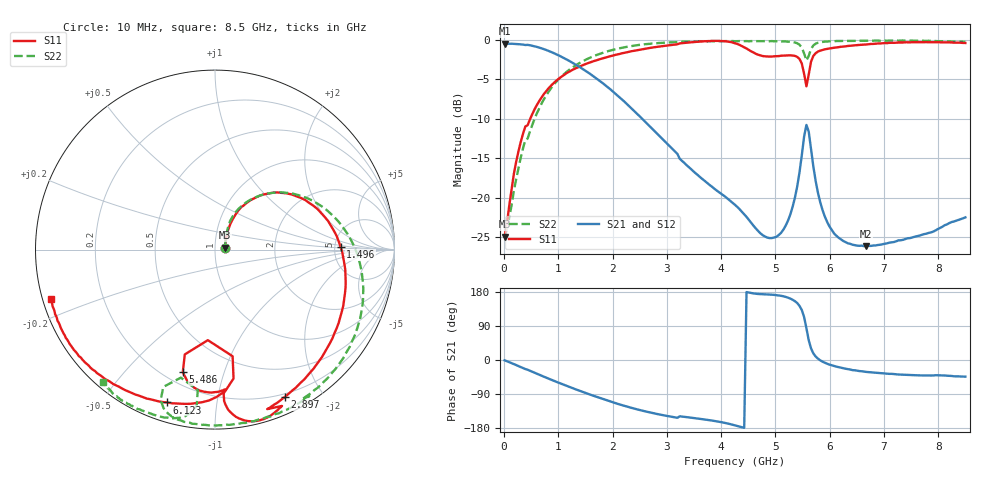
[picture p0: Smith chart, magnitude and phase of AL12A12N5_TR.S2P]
!AVX CORPORATION
!PART NUMBER AL12A12N5_TR
!DESCRIPTION: AIR CORE INDUCTOR, 12.5nH, 4 TURNS
!Agilent Technologies,E5071C,MY46102230,A.09.54
!Date: Mon Sep 03 15:48:47 2012
!Data & Calibration Information:
!Freq	S11:SOLT2(ON)	S21:SOLT2(ON)	S12:SOLT2(ON)	S22:SOLT2(ON)
# Hz S RI R 50
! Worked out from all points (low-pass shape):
!   201 points, 10 MHz to 8.5 GHz, reference 50 ohm
!   highest |S21| = -0.50 dB at 10 MHz (marker M1); lowest = -26.2 dB at 6.675 GHz (marker M2)
!   |S21| within 3 dB of the highest: start of sweep to 1.4 GHz
!   lowest |S11| = -25.0 dB at 10 MHz (marker M3), VSWR 1.12, Z = 55.9 + j1.16 ohm
!   |S11| at or under -10 dB: start of sweep to 483.2 MHz
!   |S22| runs from -24.9 to -0.1 dB; largest |S21 - S12| = 0.02
!   S11 on the Smith chart (normalised r, x): 10 MHz: 1.12, +0.02; 1.496 GHz: 5.64, +0.35; 2.897 GHz: 0.17, -1.56; 5.486 GHz: 0.27, -0.74; 6.123 GHz: 0.09, -0.73; 8.5 GHz: 0.02, -0.15
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1e7  0.0555 0.0103  0.9443 -0.0144  0.9353 0.00333  0.056 0.00982
1.798e8  0.0763 0.1184  0.9239 -0.1759  0.9254 -0.1758  0.0642 0.0892
3.9205e8  0.1488 0.2395  0.8464 -0.3745  0.8475 -0.3763  0.1107 0.2039
9.0145e8  0.4271 0.3075  0.486 -0.6685  0.4857 -0.6695  0.4011 0.3162
1.4533e9  0.6888 0.047  0.0634 -0.6477  0.0625 -0.6483  0.7229 0.11
1.49575e9  0.6998 0.0159  0.0372 -0.6357  0.0367 -0.636  0.7396 0.0857
2.09005e9  0.6782 -0.4372  -0.1912 -0.4001  -0.1912 -0.4003  0.8223 -0.3051
2.85415e9  0.4028 -0.8097  -0.1985 -0.1468  -0.1986 -0.1466  0.6223 -0.7215
2.8966e9  0.3877 -0.8219  -0.195 -0.1376  -0.1952 -0.1378  0.605 -0.7376
3.70315e9  0.3001 -0.9305  -0.1169 -0.0495  -0.1171 -0.0494  0.3562 -0.912
4.255e9  0.1335 -0.9405  -0.0891 -0.0118  -0.0891 -0.0117  0.1548 -0.9655
5.0191e9  0.0421 -0.7848  -0.0558 0.00866  -0.0558 0.00875  -0.1093 -0.9712
5.2738e9  -0.0373 -0.7955  -0.0743 0.024  -0.0742 0.024  -0.2046 -0.9481
5.48605e9  -0.1795 -0.6835  -0.1235 0.1383  -0.1232 0.1385  -0.3028 -0.8392
5.57095e9  -0.0398 -0.5046  0.0318 0.2867  0.0319 0.2864  -0.1904 -0.7134
5.6134e9  0.0981 -0.594  0.1603 0.2068  0.1604 0.2066  -0.096 -0.7834
5.6983e9  0.0584 -0.7865  0.1503 0.0475  0.1502 0.0474  -0.1357 -0.9094
5.8681e9  -0.104 -0.8549  0.0829 -0.00645  0.083 -0.00644  -0.2346 -0.94
6.1228e9  -0.2672 -0.8518  0.0546 -0.0172  0.0548 -0.0172  -0.3145 -0.9294
6.67465e9  -0.536 -0.7633  0.042 -0.0257  0.042 -0.0255  -0.4239 -0.8892
7.09915e9  -0.6834 -0.6672  0.0416 -0.0309  0.0415 -0.0306  -0.4866 -0.86
8.5e9  -0.9133 -0.2726  0.0539 -0.0519  0.054 -0.0515  -0.6255 -0.7384
